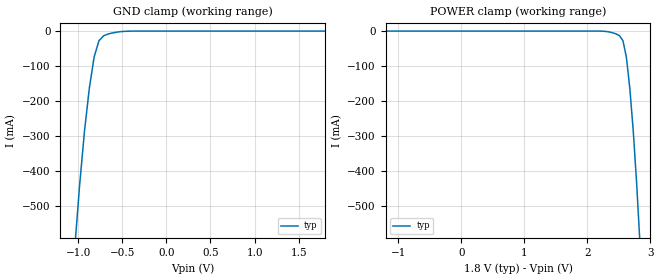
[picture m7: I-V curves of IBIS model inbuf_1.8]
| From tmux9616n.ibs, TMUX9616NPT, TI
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| inbuf_1.8
[Model]   inbuf_1.8
Model_type   Input
Vinl = 0.54
Vinh = 1.08
|   typ   min   max
C_comp   1.598234e-12   NA   NA
[Voltage Range]   1.8   NA   NA
[Temperature Range]   27   NA   NA
[Power Clamp Reference]   1.8   NA   NA
[GND Clamp Reference]   0   NA   NA
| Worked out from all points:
|   GND clamp passes 1 mA (typ) near -0.49 V on its own axis
[GND Clamp]
|   Voltage   I(typ)   I(min)   I(max)
-3.6V     -11.61A    NA         NA
-1.036V   -614.5mA   NA         NA
-981.8mV  -436.6mA   NA         NA
-927.3mV  -284.5mA   NA         NA
-872.7mV  -163.1mA   NA         NA
-818.2mV  -73.86mA   NA         NA
-763.6mV  -27.46mA   NA         NA
-709.1mV  -13.11mA   NA         NA
-600mV    -4.747mA   NA         NA
-436.4mV  -298uA     NA         NA
1.8V      189.7nA    NA         NA
[POWER Clamp]
|   Voltage   I(typ)   I(min)   I(max)
-1.8V     379.4nA    NA         NA
2.182V    -68.37uA   NA         NA
2.345V    -2.448mA   NA         NA
2.509V    -13.11mA   NA         NA
2.564V    -27.46mA   NA         NA
2.618V    -73.86mA   NA         NA
2.673V    -163.1mA   NA         NA
2.727V    -284.5mA   NA         NA
2.782V    -436.6mA   NA         NA
2.836V    -614.5mA   NA         NA
3.6V      -3.616A    NA         NA
